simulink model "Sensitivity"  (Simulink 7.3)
settings: Solver=ode5  StartTime=0.0  StopTime=100  FixedStep=Ts  RelTol=1e-3
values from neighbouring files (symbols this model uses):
  Ts = 0.04    [run.m]    (also in z2s_transf.m)
undefined symbols (not defined in the file or in its folder): Alfc, Apfc, Azpl, Blfc, Bpfc, Bzpl, Clfc, Cpfc, Czpl, Dlfc, Dpfc, Dzpl, TVC

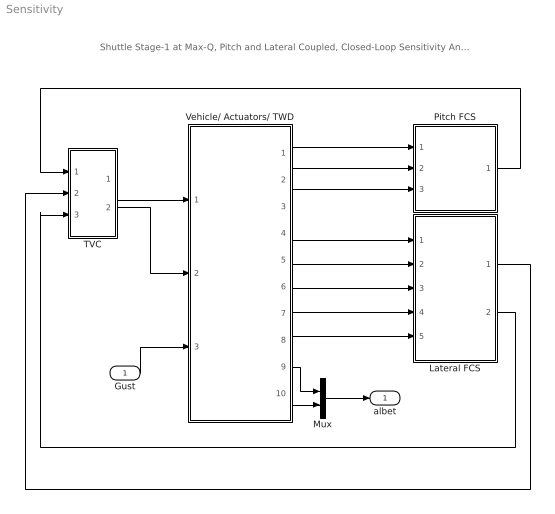
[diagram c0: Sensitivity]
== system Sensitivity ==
  note: Shuttle Stage-1 at Max-Q, Pitch and Lateral Coupled, Closed-Loop Sensitivity Analysis Model
  Gust : Inport  OutDataType=sfix(16)  OutScaling=2^0
  Lateral FCS : Subsystem
  Mux : Mux  Inputs=2
  Pitch FCS : Subsystem
  TVC : Subsystem
  Vehicle/ Actuators/ TWD : Subsystem
  albet : Outport  OutDataType=sfix(16)  OutScaling=2^0
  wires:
  Pitch FCS/1(DQ_TVC) -> TVC/1(ptch)
  Lateral FCS/1(DP_TVC) -> TVC/2(roll)
  Lateral FCS/2(DR_TVC) -> TVC/3(yaw)
  TVC/2(dz) -> Vehicle/ Actuators/ TWD/2(dzc)
  TVC/1(dy) -> Vehicle/ Actuators/ TWD/1(dyc)
  Gust/1 -> Vehicle/ Actuators/ TWD/3(WG)
  Vehicle/ Actuators/ TWD/1(theta) -> Pitch FCS/1(theta)
  Vehicle/ Actuators/ TWD/2(q-flx) -> Pitch FCS/2(q)
  Vehicle/ Actuators/ TWD/3(Nz) -> Pitch FCS/3(Nz)
  Vehicle/ Actuators/ TWD/4(phi) -> Lateral FCS/1(phi-er)
  Vehicle/ Actuators/ TWD/5(psi) -> Lateral FCS/2(psi-er)
  Vehicle/ Actuators/ TWD/6(p-flx) -> Lateral FCS/3(p)
  Vehicle/ Actuators/ TWD/7(r-flx) -> Lateral FCS/4(r)
  Vehicle/ Actuators/ TWD/8(Ny) -> Lateral FCS/5(Ny)
  Vehicle/ Actuators/ TWD/9(alfa) -> Mux/1
  Vehicle/ Actuators/ TWD/10(beta) -> Mux/2
  Mux/1 -> albet/1

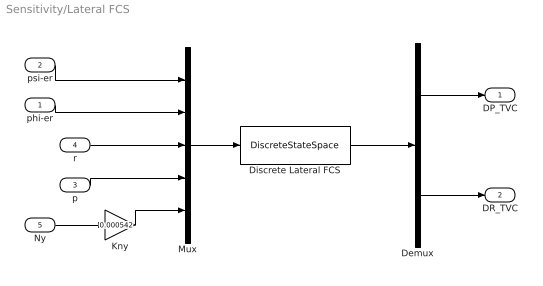
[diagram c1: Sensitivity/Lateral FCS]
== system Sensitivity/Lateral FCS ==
  phi-er : Inport  OutDataType=sfix(16)  OutScaling=2^0
  psi-er : Inport  Port=2  OutDataType=sfix(16)  OutScaling=2^0
  p : Inport  Port=3  OutDataType=sfix(16)  OutScaling=2^0
  r : Inport  Port=4  OutDataType=sfix(16)  OutScaling=2^0
  Ny : Inport  Port=5  OutDataType=sfix(16)  OutScaling=2^0
  Demux : Demux  Outputs=2
  Discrete Lateral FCS : DiscreteStateSpace  A=Alfc  B=Blfc  C=Clfc  D=Dlfc  SampleTime=Ts
  Kny : Gain  Gain=0.000542  ParameterDataType=sfix(16)  ParameterScaling=2^0  OutDataType=sfix(16)  OutScaling=2^0
  Mux : Mux  Inputs=5
  DP_TVC : Outport  OutDataType=sfix(16)  OutScaling=2^0
  DR_TVC : Outport  Port=2  OutDataType=sfix(16)  OutScaling=2^0
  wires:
  psi-er/1 -> Mux/1
  phi-er/1 -> Mux/2
  r/1 -> Mux/3
  Mux/1 -> Discrete Lateral FCS/1
  Discrete Lateral FCS/1 -> Demux/1
  Demux/1 -> DP_TVC/1
  Demux/2 -> DR_TVC/1
  p/1 -> Mux/4
  Ny/1 -> Kny/1
  Kny/1 -> Mux/5

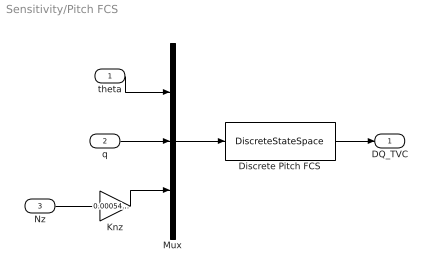
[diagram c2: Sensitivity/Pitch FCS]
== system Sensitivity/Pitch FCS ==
  theta : Inport  OutDataType=sfix(16)  OutScaling=2^0
  q : Inport  Port=2  OutDataType=sfix(16)  OutScaling=2^0
  Nz : Inport  Port=3  OutDataType=sfix(16)  OutScaling=2^0
  Discrete Pitch FCS : DiscreteStateSpace  A=Apfc  B=Bpfc  C=Cpfc  D=Dpfc  SampleTime=Ts
  Knz : Gain  Gain=0.000542*0.5  ParameterDataType=sfix(16)  ParameterScaling=2^0  OutDataType=sfix(16)  OutScaling=2^0
  Mux : Mux  Inputs=3
  DQ_TVC : Outport  OutDataType=sfix(16)  OutScaling=2^0
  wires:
  Mux/1 -> Discrete Pitch FCS/1
  Nz/1 -> Knz/1
  q/1 -> Mux/2
  theta/1 -> Mux/1
  Discrete Pitch FCS/1 -> DQ_TVC/1
  Knz/1 -> Mux/3

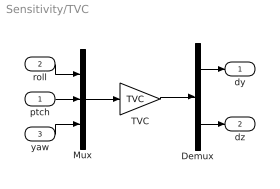
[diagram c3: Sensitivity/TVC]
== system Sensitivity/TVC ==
  ptch : Inport  OutDataType=sfix(16)  OutScaling=2^0
  roll : Inport  Port=2  OutDataType=sfix(16)  OutScaling=2^0
  yaw : Inport  Port=3  OutDataType=sfix(16)  OutScaling=2^0
  Demux : Demux  Outputs="[5  5]"
  Mux : Mux  Inputs=3
  TVC : Gain  Gain=TVC  Multiplication=Matrix(K*u) (u vector)  ParameterDataType=sfix(16)  ParameterScaling=2^0  OutDataType=sfix(16)  OutScaling=2^0
  dy : Outport  OutDataType=sfix(16)  OutScaling=2^0
  dz : Outport  Port=2  OutDataType=sfix(16)  OutScaling=2^0
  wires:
  TVC/1 -> Demux/1
  Mux/1 -> TVC/1
  roll/1 -> Mux/1
  Demux/1 -> dy/1
  ptch/1 -> Mux/2
  Demux/2 -> dz/1
  yaw/1 -> Mux/3

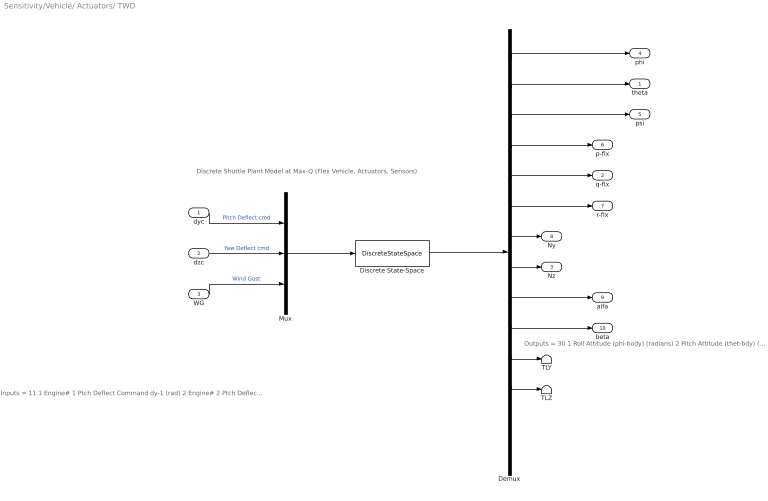
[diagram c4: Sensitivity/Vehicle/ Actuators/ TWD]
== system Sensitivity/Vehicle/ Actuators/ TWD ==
  note: Discrete Shuttle Plant Model at Max-Q (Flex Vehicle, Actuators, Sensors)
  note: Inputs = 11 1 Engine# 1 Ptch Deflect Command dy-1 (rad) 2 Engine# 2 Ptch Deflect Command dy-2 (rad) 3 Engine# 3 Ptch Deflect Command dy-3 (rad) 4 Engine# 4 Ptch Deflect Command dy-4 (rad) 5 Engine# 5 Ptch Deflect Command dy-5 (rad) 6 Engine# 1 Yaw Deflect Command dz-1 (rad) 7 Engine# 2 Yaw Deflect Command dz-2 (rad) 8 Engine# 3 Yaw Deflect Command dz-3 (rad) 9 Engine# 4 Yaw Deflect Command dz-4 (rad) 10 Engine# 5 Yaw Deflect Command dz-5 (rad) 11 Wind Gust Velocity (ft/sec)
  note: Outputs = 30 1 Roll Attitude (phi-body) (radians) 2 Pitch Attitude (thet-bdy) (radians) 3 Yaw Attitude (psi-body) (radians) 4 Roll Rate Gyro (p-flex) (rad/sec) 5 Pitch Rate Gyro (q-flex) (rad/sec) 6 Yaw Rate Gyro (r-flex) (rad/sec) 7 Accelerom # 1, Y-ddot Accelerat. (ft/sec^2) 8 Accelerom # 2, Z-ddot Accelerat. (ft/sec^2) 9 Angle of attack, alfa, (radians) 10 Angle of sideslip, beta, (radian) 11 Load-Torque Pitch TLY-Eng-1 12 Load-Torque Pitch TLY-Eng-2 13 Load-Torque Pitch TLY-Eng-3 14 Load-Torque Pitch TLY-Eng-4 15 Load-Torque Pitch TLY-Eng-5 16 Load-Torque Yaw TLZ-Eng-1 17 Load-Torque Yaw TLZ-Eng-2 18 Load-Torque Yaw TLZ-Eng-3 19 Load-Torque Yaw TLZ-Eng-4 20 Load-Torque Yaw TLZ-Eng-5 21 Engine # 1 Pitch Deflection dy-1 (rad) 22 Engine # 2 Pitch Deflection dy-2 (rad) 23 Engine # 3 Pitch Deflection dy-3 (rad) 24 Engine # 4 Pitch Deflection dy-4 (rad) 25 Engine # 5 Pitch Deflection dy-5 (rad) 26 Engine # 1 Yaw Deflection dz-1 (rad) 27 Engine # 2 Yaw Deflection dz-2 (rad) 28 Engine # 3 Yaw Deflection dz-3 (rad) 29 Engine # 4 Yaw Deflection dz-4 (rad) 30 Engine # 5 Yaw Deflection dz-5 (rad)
  dyc : Inport  PortDimensions=5  OutDataType=sfix(16)  OutScaling=2^0
  dzc : Inport  Port=2  PortDimensions=5  OutDataType=sfix(16)  OutScaling=2^0
  WG : Inport  Port=3  OutDataType=sfix(16)  OutScaling=2^0
  Demux : Demux  Outputs=[1,1,1,1,1,1,1,1,1,1, 5,5,5,5]
  Discrete State-Space : DiscreteStateSpace  A=Azpl  B=Bzpl  C=Czpl  D=Dzpl  SampleTime=Ts
  Mux : Mux  Inputs="[5  5  1]"
  TLY : Terminator
  TLZ : Terminator
  theta : Outport  OutDataType=sfix(16)  OutScaling=2^0
  q-flx : Outport  Port=2  OutDataType=sfix(16)  OutScaling=2^0
  Nz : Outport  Port=3  OutDataType=sfix(16)  OutScaling=2^0
  phi : Outport  Port=4  OutDataType=sfix(16)  OutScaling=2^0
  psi : Outport  Port=5  OutDataType=sfix(16)  OutScaling=2^0
  p-flx : Outport  Port=6  OutDataType=sfix(16)  OutScaling=2^0
  r-flx : Outport  Port=7  OutDataType=sfix(16)  OutScaling=2^0
  Ny : Outport  Port=8  OutDataType=sfix(16)  OutScaling=2^0
  alfa : Outport  Port=9  OutDataType=sfix(16)  OutScaling=2^0
  beta : Outport  Port=10  OutDataType=sfix(16)  OutScaling=2^0
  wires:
  dyc/1 -> Mux/1  "Pitch Deflect cmd"
  dzc/1 -> Mux/2  "Yaw Deflect cmd"
  WG/1 -> Mux/3  "Wind Gust"
  Mux/1 -> Discrete State-Space/1
  Discrete State-Space/1 -> Demux/1
  Demux/1 -> phi/1
  Demux/2 -> theta/1
  Demux/3 -> psi/1
  Demux/4 -> p-flx/1
  Demux/5 -> q-flx/1
  Demux/6 -> r-flx/1
  Demux/7 -> Ny/1
  Demux/8 -> Nz/1
  Demux/9 -> alfa/1
  Demux/10 -> beta/1
  Demux/11 -> TLY/1
  Demux/12 -> TLZ/1
